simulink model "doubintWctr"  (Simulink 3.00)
settings: Solver=ode45  StartTime=0.0  StopTime=100  RelTol=1e-3
libraries: simulink3 x1

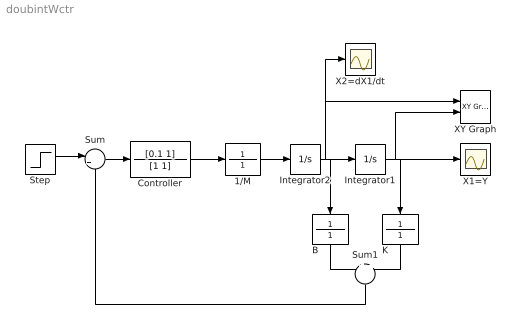
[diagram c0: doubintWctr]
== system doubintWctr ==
  1/M : TransferFcn  Numerator=1  Denominator=1
  B : TransferFcn  Orientation=down  Numerator=1  Denominator=1
  Controller : TransferFcn  Numerator=[0.1 1]  Denominator=[1 1]
  Integrator1 : Integrator  ExternalReset=none  InitialConditionSource=internal  InitialCondition=0  LimitOutput=off  UpperSaturationLimit=inf  LowerSaturationLimit=-inf  ShowSaturationPort=off  ShowStatePort=off  AbsoluteTolerance=auto
  Integrator2 : Integrator  ExternalReset=none  InitialConditionSource=internal  InitialCondition=0  LimitOutput=off  UpperSaturationLimit=inf  LowerSaturationLimit=-inf  ShowSaturationPort=off  ShowStatePort=off  AbsoluteTolerance=auto
  K : TransferFcn  Tag=K  Orientation=down  Numerator=1  Denominator=1
  Step : Step  Time=0  Before=0  After=1  SampleTime=0
  Sum : Sum  Inputs=|+-  SaturateOnIntegerOverflow=on
  Sum1 : Sum  Orientation=down  Inputs=+||+  SaturateOnIntegerOverflow=on
  X1=Y : Scope
  X2=dX1/dt : Scope
  XY Graph : simulink3/Sinks/XY Graph  xmin=-1  xmax=1  ymin=-1  ymax=2  st=.1
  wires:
  Step/1 -> Sum/1
  Sum/1 -> Controller/1
  Sum1/1 -> Sum/2
  Integrator1/1 -> X1=Y/1, K/1, XY Graph/2
  1/M/1 -> Integrator2/1
  Integrator2/1 -> Integrator1/1, B/1, X2=dX1/dt/1, XY Graph/1
  Controller/1 -> 1/M/1
  K/1 -> Sum1/2
  B/1 -> Sum1/1
